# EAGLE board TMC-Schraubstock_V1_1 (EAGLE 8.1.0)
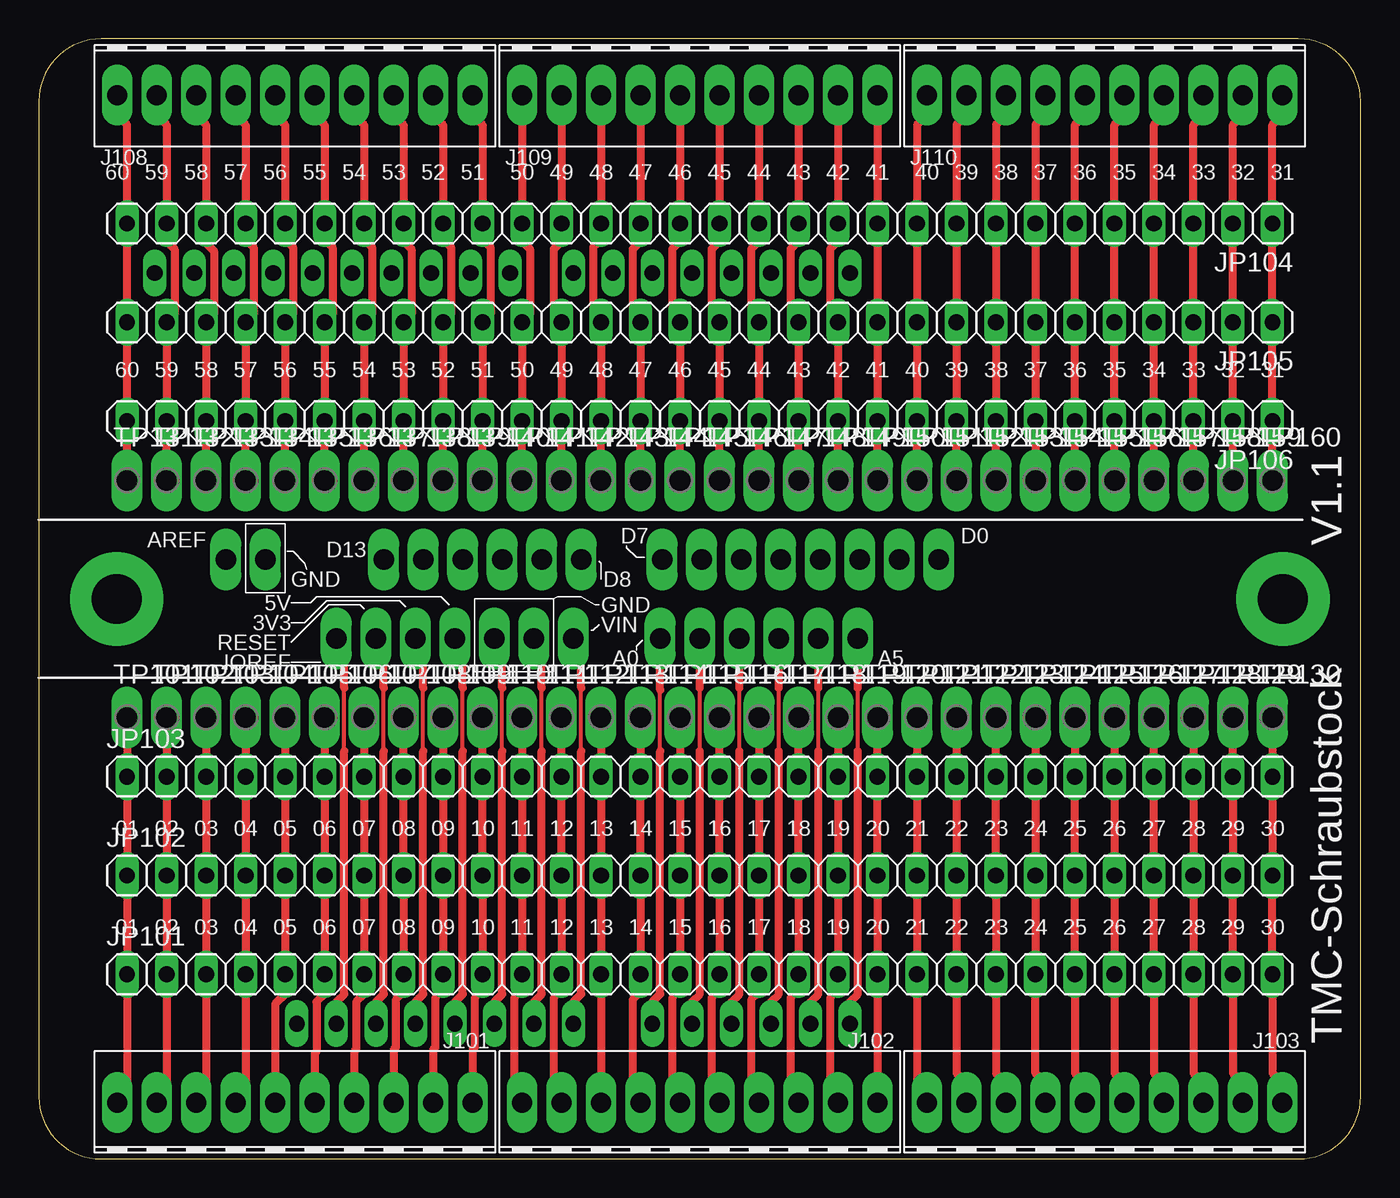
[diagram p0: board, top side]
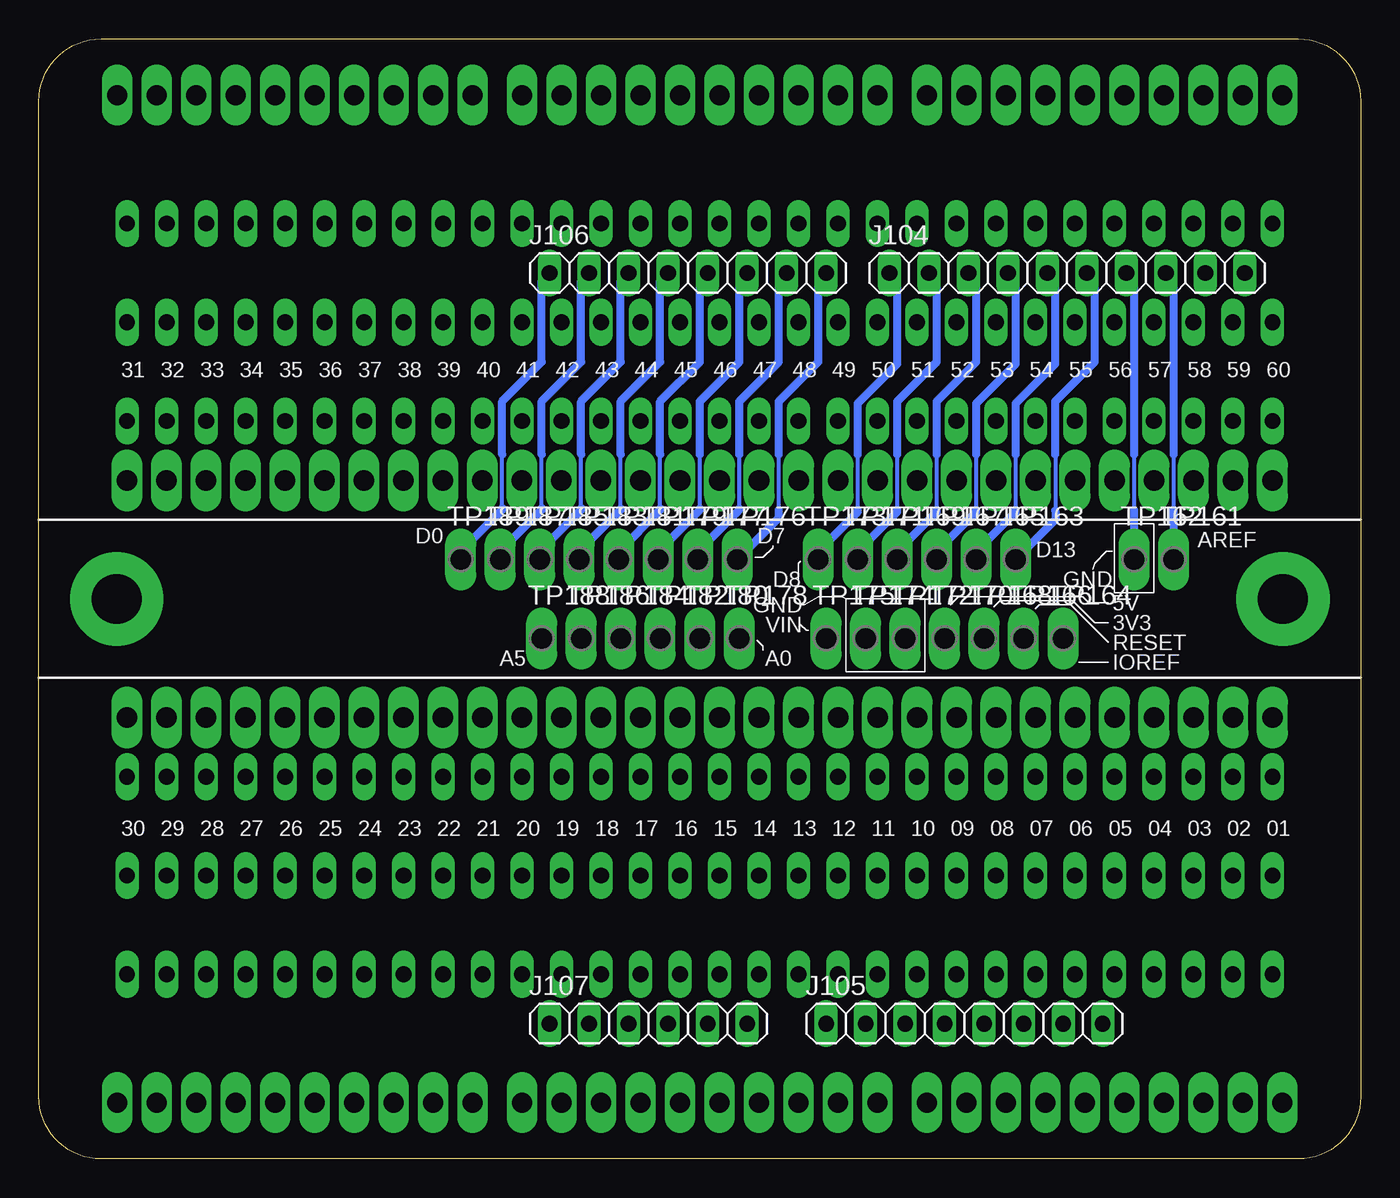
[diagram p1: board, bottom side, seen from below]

Size 85 x 72 mm. Coordinates in mm from the lower left corner, seen from the top.
Outline: 0,68 0,4 arc90 4,0 81,0 arc90 85,4 85,68 arc90 81,72 4,72 arc90 0,68
Copper layers (1*16): Top 0.018mm / dielectric 1.55mm / Bottom 0.018mm
Design rules "eC_2Layer_PClass6_BaseCopperO18_eCDefault": minimum track width 0.15mm, minimum drill 0.35mm, track to track 0.15mm, track to pad 0.15mm, pad to pad 0.15mm, via to via 0.15mm, smd to smd 0mil, copper to edge 0.25mm, drill to drill 0.35mm, minimum pad ring 0.175mm, minimum via ring 0.125mm, stop-mask expansion 0mil, vias tented up to drill 0.45mm, thermal gap 0.2mm

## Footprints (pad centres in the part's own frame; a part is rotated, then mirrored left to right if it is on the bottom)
OSTVN10A150 = drill 1.3 long: 1 -11.43,0; 2 -8.89,0; 3 -6.35,0; 4 -3.81,0; 5 -1.27,0; 6 1.27,0; 7 3.81,0; 8 6.35,0; 9 8.89,0; 10 11.43,0
1X10 = drill 1.016 long: 1 -11.43,0; 2 -8.89,0; 3 -6.35,0; 4 -3.81,0; 5 -1.27,0; 6 1.27,0; 7 3.81,0; 8 6.35,0; 9 8.89,0; 10 11.43,0
1X08 = drill 1.016 long: 1 -8.89,0; 2 -6.35,0; 3 -3.81,0; 4 -1.27,0; 5 1.27,0; 6 3.81,0; 7 6.35,0; 8 8.89,0
1X06 = drill 1.016 long: 1 -6.35,0; 2 -3.81,0; 3 -1.27,0; 4 1.27,0; 5 3.81,0; 6 6.35,0
1X30 = drill 1.016 long: 1 -36.83,0; 2 -34.29,0; 3 -31.75,0; 4 -29.21,0; 5 -26.67,0; 6 -24.13,0; 7 -21.59,0; 8 -19.05,0; 9 -16.51,0; 10 -13.97,0; 11 -11.43,0; 12 -8.89,0; 13 -6.35,0; 14 -3.81,0; 15 -1.27,0; 16 1.27,0; 17 3.81,0; 18 6.35,0; 19 8.89,0; 20 11.43,0; 21 13.97,0; 22 16.51,0; 23 19.05,0; 24 21.59,0; 25 24.13,0; 26 26.67,0; 27 29.21,0; 28 31.75,0; 29 34.29,0; 30 36.83,0
P1-13Y = drill 1.321 pad 1.905 long: TP 0,0

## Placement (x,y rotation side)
J101  [OSTVN10A150]  16.46,3.62 0 top
J102  [OSTVN10A150]  42.5,3.62 0 top
J103  [OSTVN10A150]  68.53,3.62 0 top
J104  PINHD-1X10  [1X10]  18.88,56.95 0 bottom
J105  PINHD-1X8  [1X08]  25.48,8.7 0 bottom
J106  PINHD-1X8  [1X08]  43.26,56.95 0 bottom
J107  PINHD-1X6  [1X06]  45.8,8.7 0 bottom
J108  [OSTVN10A150]  16.46,68.38 180 top
J109  [OSTVN10A150]  42.5,68.38 180 top
J110  [OSTVN10A150]  68.53,68.38 180 top
JP101  [1X30]  42.5,11.87 0 top
JP102  [1X30]  42.5,18.22 0 top
JP103  [1X30]  42.5,24.57 0 top
JP104  [1X30]  42.5,60.13 180 top
JP105  [1X30]  42.5,53.78 180 top
JP106  [1X30]  42.5,47.43 180 top
TP101  TPSPAD1-13Y  [P1-13Y]  5.67,28.38 0 top
TP102  TPSPAD1-13Y  [P1-13Y]  8.21,28.38 0 top
TP103  TPSPAD1-13Y  [P1-13Y]  10.75,28.38 0 top
TP104  TPSPAD1-13Y  [P1-13Y]  13.29,28.38 0 top
TP105  TPSPAD1-13Y  [P1-13Y]  15.83,28.38 0 top
TP106  TPSPAD1-13Y  [P1-13Y]  18.37,28.38 0 top
TP107  TPSPAD1-13Y  [P1-13Y]  20.91,28.38 0 top
TP108  TPSPAD1-13Y  [P1-13Y]  23.45,28.38 0 top
TP109  TPSPAD1-13Y  [P1-13Y]  25.99,28.38 0 top
TP110  TPSPAD1-13Y  [P1-13Y]  28.53,28.38 0 top
TP111  TPSPAD1-13Y  [P1-13Y]  31.07,28.38 0 top
TP112  TPSPAD1-13Y  [P1-13Y]  33.61,28.38 0 top
TP113  TPSPAD1-13Y  [P1-13Y]  36.15,28.38 0 top
TP114  TPSPAD1-13Y  [P1-13Y]  38.69,28.38 0 top
TP115  TPSPAD1-13Y  [P1-13Y]  41.23,28.38 0 top
TP116  TPSPAD1-13Y  [P1-13Y]  43.77,28.38 0 top
TP117  TPSPAD1-13Y  [P1-13Y]  46.31,28.38 0 top
TP118  TPSPAD1-13Y  [P1-13Y]  48.85,28.38 0 top
TP119  TPSPAD1-13Y  [P1-13Y]  51.39,28.38 0 top
TP120  TPSPAD1-13Y  [P1-13Y]  53.93,28.38 0 top
TP121  TPSPAD1-13Y  [P1-13Y]  56.47,28.38 0 top
TP122  TPSPAD1-13Y  [P1-13Y]  59.01,28.38 0 top
TP123  TPSPAD1-13Y  [P1-13Y]  61.55,28.38 0 top
TP124  TPSPAD1-13Y  [P1-13Y]  64.09,28.38 0 top
TP125  TPSPAD1-13Y  [P1-13Y]  66.63,28.38 0 top
TP126  TPSPAD1-13Y  [P1-13Y]  69.17,28.38 0 top
TP127  TPSPAD1-13Y  [P1-13Y]  71.71,28.38 0 top
TP128  TPSPAD1-13Y  [P1-13Y]  74.25,28.38 0 top
TP129  TPSPAD1-13Y  [P1-13Y]  76.79,28.38 0 top
TP130  TPSPAD1-13Y  [P1-13Y]  79.33,28.38 0 top
TP131  TPSPAD1-13Y  [P1-13Y]  5.67,43.62 0 top
TP132  TPSPAD1-13Y  [P1-13Y]  8.21,43.62 0 top
TP133  TPSPAD1-13Y  [P1-13Y]  10.75,43.62 0 top
TP134  TPSPAD1-13Y  [P1-13Y]  13.29,43.62 0 top
TP135  TPSPAD1-13Y  [P1-13Y]  15.83,43.62 0 top
TP136  TPSPAD1-13Y  [P1-13Y]  18.37,43.62 0 top
TP137  TPSPAD1-13Y  [P1-13Y]  20.91,43.62 0 top
TP138  TPSPAD1-13Y  [P1-13Y]  23.45,43.62 0 top
TP139  TPSPAD1-13Y  [P1-13Y]  25.99,43.62 0 top
TP140  TPSPAD1-13Y  [P1-13Y]  28.53,43.62 0 top
TP141  TPSPAD1-13Y  [P1-13Y]  31.07,43.62 0 top
TP142  TPSPAD1-13Y  [P1-13Y]  33.61,43.62 0 top
TP143  TPSPAD1-13Y  [P1-13Y]  36.15,43.62 0 top
TP144  TPSPAD1-13Y  [P1-13Y]  38.69,43.62 0 top
TP145  TPSPAD1-13Y  [P1-13Y]  41.23,43.62 0 top
TP146  TPSPAD1-13Y  [P1-13Y]  43.77,43.62 0 top
TP147  TPSPAD1-13Y  [P1-13Y]  46.31,43.62 0 top
TP148  TPSPAD1-13Y  [P1-13Y]  48.85,43.62 0 top
TP149  TPSPAD1-13Y  [P1-13Y]  51.39,43.62 0 top
TP150  TPSPAD1-13Y  [P1-13Y]  53.93,43.62 0 top
TP151  TPSPAD1-13Y  [P1-13Y]  56.47,43.62 0 top
TP152  TPSPAD1-13Y  [P1-13Y]  59.01,43.62 0 top
TP153  TPSPAD1-13Y  [P1-13Y]  61.55,43.62 0 top
TP154  TPSPAD1-13Y  [P1-13Y]  64.09,43.62 0 top
TP155  TPSPAD1-13Y  [P1-13Y]  66.63,43.62 0 top
TP156  TPSPAD1-13Y  [P1-13Y]  69.17,43.62 0 top
TP157  TPSPAD1-13Y  [P1-13Y]  71.71,43.62 0 top
TP158  TPSPAD1-13Y  [P1-13Y]  74.25,43.62 0 top
TP159  TPSPAD1-13Y  [P1-13Y]  76.79,43.62 0 top
TP160  TPSPAD1-13Y  [P1-13Y]  79.33,43.62 0 top
TP161  TPSPAD1-13Y  [P1-13Y]  12.02,38.54 0 bottom
TP162  TPSPAD1-13Y  [P1-13Y]  14.56,38.54 0 bottom
TP163  TPSPAD1-13Y  [P1-13Y]  22.18,38.54 0 bottom
TP164  TPSPAD1-13Y  [P1-13Y]  19.13,33.46 0 bottom
TP165  TPSPAD1-13Y  [P1-13Y]  24.72,38.54 0 bottom
TP166  TPSPAD1-13Y  [P1-13Y]  21.67,33.46 0 bottom
TP167  TPSPAD1-13Y  [P1-13Y]  27.26,38.54 0 bottom
TP168  TPSPAD1-13Y  [P1-13Y]  24.21,33.46 0 bottom
TP169  TPSPAD1-13Y  [P1-13Y]  29.8,38.54 0 bottom
TP170  TPSPAD1-13Y  [P1-13Y]  26.75,33.46 0 bottom
TP171  TPSPAD1-13Y  [P1-13Y]  32.34,38.54 0 bottom
TP172  TPSPAD1-13Y  [P1-13Y]  29.29,33.46 0 bottom
TP173  TPSPAD1-13Y  [P1-13Y]  34.88,38.54 0 bottom
TP174  TPSPAD1-13Y  [P1-13Y]  31.83,33.46 0 bottom
TP175  TPSPAD1-13Y  [P1-13Y]  34.37,33.46 0 bottom
TP176  TPSPAD1-13Y  [P1-13Y]  40.09,38.54 0 bottom
TP177  TPSPAD1-13Y  [P1-13Y]  42.63,38.54 0 bottom
TP178  TPSPAD1-13Y  [P1-13Y]  39.96,33.46 0 bottom
TP179  TPSPAD1-13Y  [P1-13Y]  45.17,38.54 0 bottom
TP180  TPSPAD1-13Y  [P1-13Y]  42.5,33.46 0 bottom
TP181  TPSPAD1-13Y  [P1-13Y]  47.71,38.54 0 bottom
TP182  TPSPAD1-13Y  [P1-13Y]  45.04,33.46 0 bottom
TP183  TPSPAD1-13Y  [P1-13Y]  50.25,38.54 0 bottom
TP184  TPSPAD1-13Y  [P1-13Y]  47.58,33.46 0 bottom
TP185  TPSPAD1-13Y  [P1-13Y]  52.79,38.54 0 bottom
TP186  TPSPAD1-13Y  [P1-13Y]  50.12,33.46 0 bottom
TP187  TPSPAD1-13Y  [P1-13Y]  55.33,38.54 0 bottom
TP188  TPSPAD1-13Y  [P1-13Y]  52.66,33.46 0 bottom
TP189  TPSPAD1-13Y  [P1-13Y]  57.87,38.54 0 bottom

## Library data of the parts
J101-J110 TP101-TP189 = TMC-Schraubstock
JP101-JP106 = pinhead

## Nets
N$1: J101.1 JP101.1 JP102.1 JP103.1 TP101.TP
N$2: J101.2 JP101.2 JP102.2 JP103.2 TP102.TP
N$3: J101.3 JP101.3 JP102.3 JP103.3 TP103.TP
N$4: J101.4 JP101.4 JP102.4 JP103.4 TP104.TP
N$5: J101.5 JP101.5 JP102.5 JP103.5 TP105.TP
N$6: J101.6 JP101.6 JP102.6 JP103.6 TP106.TP
N$7: J101.7 JP101.7 JP102.7 JP103.7 TP107.TP
N$8: J101.8 JP101.8 JP102.8 JP103.8 TP108.TP
N$9: J101.9 JP101.9 JP102.9 JP103.9 TP109.TP
N$10: J101.10 JP101.10 JP102.10 JP103.10 TP110.TP
N$11: J102.1 JP101.11 JP102.11 JP103.11 TP111.TP
N$12: J102.2 JP101.12 JP102.12 JP103.12 TP112.TP
N$13: J102.3 JP101.13 JP102.13 JP103.13 TP113.TP
N$14: J102.4 JP101.14 JP102.14 JP103.14 TP114.TP
N$15: J102.5 JP101.15 JP102.15 JP103.15 TP115.TP
N$16: J102.6 JP101.16 JP102.16 JP103.16 TP116.TP
N$17: J102.7 JP101.17 JP102.17 JP103.17 TP117.TP
N$18: J102.8 JP101.18 JP102.18 JP103.18 TP118.TP
N$19: J102.9 JP101.19 JP102.19 JP103.19 TP119.TP
N$20: J102.10 JP101.20 JP102.20 JP103.20 TP120.TP
N$21: J103.1 JP101.21 JP102.21 JP103.21 TP121.TP
N$22: J103.2 JP101.22 JP102.22 JP103.22 TP122.TP
N$23: J103.3 JP101.23 JP102.23 JP103.23 TP123.TP
N$24: J103.4 JP101.24 JP102.24 JP103.24 TP124.TP
N$25: J103.5 JP101.25 JP102.25 JP103.25 TP125.TP
N$26: J103.6 JP101.26 JP102.26 JP103.26 TP126.TP
N$27: J103.7 JP101.27 JP102.27 JP103.27 TP127.TP
N$28: J103.8 JP101.28 JP102.28 JP103.28 TP128.TP
N$29: J103.9 JP101.29 JP102.29 JP103.29 TP129.TP
N$30: J103.10 JP101.30 JP102.30 JP103.30 TP130.TP
N$31: J110.1 JP104.1 JP105.1 JP106.1 TP160.TP
N$32: J110.2 JP104.2 JP105.2 JP106.2 TP159.TP
N$33: J110.3 JP104.3 JP105.3 JP106.3 TP158.TP
N$34: J110.4 JP104.4 JP105.4 JP106.4 TP157.TP
N$35: J110.5 JP104.5 JP105.5 JP106.5 TP156.TP
N$36: J110.6 JP104.6 JP105.6 JP106.6 TP155.TP
N$37: J110.7 JP104.7 JP105.7 JP106.7 TP154.TP
N$38: J110.8 JP104.8 JP105.8 JP106.8 TP153.TP
N$39: J110.9 JP104.9 JP105.9 JP106.9 TP152.TP
N$40: J110.10 JP104.10 JP105.10 JP106.10 TP151.TP
N$41: J109.1 JP104.11 JP105.11 JP106.11 TP150.TP
N$42: J109.2 JP104.12 JP105.12 JP106.12 TP149.TP
N$43: J109.3 JP104.13 JP105.13 JP106.13 TP148.TP
N$44: J109.4 JP104.14 JP105.14 JP106.14 TP147.TP
N$45: J109.5 JP104.15 JP105.15 JP106.15 TP146.TP
N$46: J109.6 JP104.16 JP105.16 JP106.16 TP145.TP
N$47: J109.7 JP104.17 JP105.17 JP106.17 TP144.TP
N$48: J109.8 JP104.18 JP105.18 JP106.18 TP143.TP
N$49: J109.9 JP104.19 JP105.19 JP106.19 TP142.TP
N$50: J109.10 JP104.20 JP105.20 JP106.20 TP141.TP
N$51: J108.1 JP104.21 JP105.21 JP106.21 TP140.TP
N$52: J108.2 JP104.22 JP105.22 JP106.22 TP139.TP
N$53: J108.3 JP104.23 JP105.23 JP106.23 TP138.TP
N$54: J108.4 JP104.24 JP105.24 JP106.24 TP137.TP
N$55: J108.5 JP104.25 JP105.25 JP106.25 TP136.TP
N$56: J108.6 JP104.26 JP105.26 JP106.26 TP135.TP
N$57: J108.7 JP104.27 JP105.27 JP106.27 TP134.TP
N$58: J108.8 JP104.28 JP105.28 JP106.28 TP133.TP
N$59: J108.9 JP104.29 JP105.29 JP106.29 TP132.TP
N$60: J108.10 JP104.30 JP105.30 JP106.30 TP131.TP
N$62: J107.1 TP188.TP
N$63: J107.2 TP186.TP
N$64: J107.3 TP184.TP
N$65: J107.4 TP182.TP
N$66: J107.5 TP180.TP
N$67: J107.6 TP178.TP
N$68: J105.1 TP175.TP
N$69: J105.2 TP174.TP
N$70: J105.3 TP172.TP
N$71: J105.4 TP170.TP
N$72: J105.5 TP168.TP
N$73: J105.6 TP166.TP
N$74: J105.7 TP164.TP
N$76: J106.8 TP176.TP
N$77: J106.7 TP177.TP
N$78: J106.6 TP179.TP
N$79: J106.5 TP181.TP
N$80: J106.4 TP183.TP
N$81: J106.3 TP185.TP
N$82: J106.2 TP187.TP
N$83: J106.1 TP189.TP
N$86: J104.8 TP161.TP
N$87: J104.7 TP162.TP
N$88: J104.6 TP163.TP
N$89: J104.5 TP165.TP
N$90: J104.4 TP167.TP
N$91: J104.3 TP169.TP
N$92: J104.2 TP171.TP
N$93: J104.1 TP173.TP

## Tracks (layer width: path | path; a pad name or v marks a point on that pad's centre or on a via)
N$1
  Top 0.508: TP101.TP JP103.1 JP102.1 JP101.1 5.67,4.25 J101.1
N$2
  Top 0.508: TP102.TP JP103.2 JP102.2 JP101.2 8.21,4.25 J101.2
N$3
  Top 0.508: TP103.TP JP103.3 JP102.3 JP101.3 10.75,4.25 J101.3
N$4
  Top 0.508: TP104.TP JP103.4 JP102.4 JP101.4 13.29,4.25 J101.4
N$5
  Top 0.508: TP105.TP JP103.5 JP102.5 JP101.5 | JP101.5 15.83,10.85 | JP101.5 15.83,10.6 15.2,9.96 J101.5
N$6
  Top 0.508: TP106.TP JP103.6 JP102.6 JP101.6 18.37,10.6 17.86,10.09 17.86,6.92 17.73,6.79 J101.6
N$7
  Top 0.508: TP107.TP JP103.7 JP102.7 JP101.7 20.91,10.6 20.4,10.09 20.4,7.04 20.27,6.92 J101.7
N$8
  Top 0.508: TP108.TP JP103.8 JP102.8 JP101.8 23.45,10.73 22.94,10.22 22.94,7.17 22.82,7.04 J101.8
N$9
  Top 0.508: TP109.TP JP103.9 JP102.9 JP101.9 25.99,10.85 25.48,10.35 25.48,7.17 25.36,7.04 J101.9
N$10
  Top 0.508: JP101.10 JP102.10 JP103.10 TP110.TP | JP101.10 28.53,11.74 | JP101.10 28.53,10.85 28.02,10.35 28.02,7.17 27.89,7.04 J101.10
N$11
  Top 0.508: TP111.TP JP103.11 JP102.11 JP101.11 31.07,10.85 30.56,10.35 30.56,4.12 J102.1
N$12
  Top 0.508: TP112.TP JP103.12 JP102.12 JP101.12 33.61,10.85 33.1,10.35 33.1,4.12 J102.2
N$13
  Top 0.508: TP113.TP JP103.13 JP102.13 JP101.13 J102.3
N$14
  Top 0.508: TP114.TP JP103.14 JP102.14 JP101.14 38.69,10.73 38.18,10.22 38.18,4.12 J102.4
N$15
  Top 0.508: TP115.TP JP103.15 41.25,24.55 41.25,18.22 JP102.15 JP101.15 41.23,10.85 40.72,10.35 40.72,4.12 J102.5
N$16
  Top 0.508: TP116.TP JP103.16 JP102.16 JP101.16 43.77,10.85 43.26,10.35 43.26,4.12 J102.6
N$17
  Top 0.508: TP117.TP JP103.17 JP102.17 JP101.17 46.31,10.73 45.8,10.22 45.8,4.12 J102.7
N$18
  Top 0.508: TP118.TP JP103.18 JP102.18 JP101.18 48.85,10.85 48.34,10.35 48.34,4.12 J102.8
N$19
  Top 0.508: TP119.TP JP103.19 JP102.19 JP101.19 51.39,10.85 50.88,10.35 50.88,4.12 J102.9
N$20
  Top 0.508: TP120.TP JP103.20 JP102.20 JP101.20 J102.10
N$21
  Top 0.508: TP121.TP JP103.21 JP102.21 JP101.21 56.47,4.25 J103.1
N$22
  Top 0.508: TP122.TP JP103.22 JP102.22 JP101.22 59.01,5.52 59.64,4.89 J103.2
N$23
  Top 0.508: TP123.TP JP103.23 JP102.23 JP101.23 61.55,5.52 62.19,4.89 J103.3
N$24
  Top 0.508: TP124.TP JP103.24 JP102.24 JP101.24 64.09,5.52 64.72,4.89 J103.4
N$25
  Top 0.508: TP125.TP JP103.25 JP102.25 JP101.25 66.63,5.52 67.27,4.89 J103.5
N$26
  Top 0.508: TP126.TP JP103.26 JP102.26 JP101.26 69.17,5.52 69.81,4.89 J103.6
N$27
  Top 0.508: TP127.TP JP103.27 JP102.27 JP101.27 71.71,5.52 72.34,4.89 J103.7
N$28
  Top 0.508: TP128.TP JP103.28 JP102.28 JP101.28 74.25,5.52 74.88,4.89 J103.8
N$29
  Top 0.508: TP129.TP JP103.29 JP102.29 JP101.29 76.79,5.52 77.42,4.89 J103.9
N$30
  Top 0.508: TP130.TP JP103.30 JP102.30 | JP102.30 79.33,17.59 | JP102.30 JP101.30 79.33,5.52 79.97,4.89 J103.10
N$31
  Top 0.508: TP160.TP JP106.1 JP105.1 JP104.1 79.33,66.48 79.97,67.11 J110.1
N$32
  Top 0.508: TP159.TP JP106.2 JP105.2 JP104.2 76.79,66.48 77.42,67.11 J110.2
N$33
  Top 0.508: TP158.TP JP106.3 JP105.3 JP104.3 74.25,66.48 74.88,67.11 J110.3
N$34
  Top 0.508: TP157.TP JP106.4 JP105.4 JP104.4 71.71,66.48 72.34,67.11 J110.4
N$35
  Top 0.508: TP156.TP JP106.5 JP105.5 JP104.5 69.17,66.48 69.81,67.11 J110.5
N$36
  Top 0.508: TP155.TP JP106.6 JP105.6 JP104.6 66.63,66.48 67.27,67.11 J110.6
N$37
  Top 0.508: TP154.TP JP106.7 JP105.7 JP104.7 64.09,66.48 64.72,67.11 J110.7
N$38
  Top 0.508: TP153.TP JP106.8 JP105.8 JP104.8 61.55,66.48 62.19,67.11 J110.8
N$39
  Top 0.508: TP152.TP JP106.9 JP105.9 JP104.9 59.01,66.48 59.64,67.11 J110.9
N$40
  Top 0.508: TP151.TP JP106.10 JP105.10 JP104.10 56.47,66.48 57.11,67.11 J110.10
N$41
  Top 0.508: J109.1 JP104.11 JP105.11 JP106.11 TP150.TP
N$42
  Top 0.508: J109.2 JP104.12 | TP149.TP JP106.12 JP105.12 50.88,54.29 50.88,58.48 51.39,58.99 JP104.12 | JP104.12 51.39,59.88
N$43
  Top 0.508: J109.3 JP104.13 | TP148.TP JP106.13 JP105.13 48.34,54.29 48.34,58.48 48.85,58.99 JP104.13 | JP104.13 48.85,60
N$44
  Top 0.508: J109.4 JP104.14 46.31,58.99 45.8,58.48 45.8,54.29 JP105.14 JP106.14 TP147.TP
N$45
  Top 0.508: TP146.TP JP106.15 JP105.15 43.26,54.29 43.26,58.48 43.77,58.99 JP104.15 J109.5
N$46
  Top 0.508: TP145.TP JP106.16 JP105.16 40.72,54.29 40.72,58.48 41.23,58.99 JP104.16 J109.6
N$47
  Top 0.508: TP144.TP JP106.17 JP105.17 38.18,54.29 38.18,58.48 38.69,58.99 JP104.17 | J109.7 JP104.17 | JP104.17 38.69,59.75
N$48
  Top 0.508: TP143.TP JP106.18 JP105.18 35.64,54.29 35.64,58.61 36.15,59.11 JP104.18 J109.8
N$49
  Top 0.508: TP142.TP JP106.19 JP105.19 33.1,54.29 33.1,58.48 33.61,58.99 JP104.19 J109.9
N$50
  Top 0.508: TP141.TP JP106.20 JP105.20 31.58,54.29 31.58,58.48 31.07,58.99 JP104.20 J109.10
N$51
  Top 0.508: TP140.TP JP106.21 JP105.21 29.04,54.29 29.04,58.61 28.53,59.11 JP104.21 28.53,66.48 27.89,67.11 J108.1
N$52
  Top 0.508: TP139.TP JP106.22 JP105.22 26.5,54.29 26.5,58.61 25.99,59.11 JP104.22 25.99,66.48 25.36,67.11 J108.2
N$53
  Top 0.508: TP138.TP JP106.23 JP105.23 23.96,54.29 23.96,58.48 23.45,58.99 JP104.23 23.45,66.48 22.82,67.11 J108.3
N$54
  Top 0.508: TP137.TP JP106.24 JP105.24 21.42,54.29 21.42,58.61 20.91,59.11 JP104.24 20.91,66.48 20.27,67.11 J108.4
N$55
  Top 0.508: TP136.TP JP106.25 JP105.25 18.88,54.29 18.88,58.61 18.37,59.11 JP104.25 18.37,66.48 17.73,67.11 J108.5
N$56
  Top 0.508: TP135.TP JP106.26 JP105.26 16.34,54.29 16.34,58.61 15.83,59.11 JP104.26 15.83,66.48 15.2,67.11 J108.6
N$57
  Top 0.508: TP134.TP JP106.27 JP105.27 13.8,54.29 13.8,58.61 13.29,59.11 JP104.27 13.29,66.48 12.66,67.11 J108.7
N$58
  Top 0.508: TP133.TP JP106.28 JP105.28 11.26,54.29 11.26,58.35 10.75,58.86 JP104.28 10.75,66.48 10.12,67.11 J108.8
N$59
  Top 0.508: TP132.TP JP106.29 JP105.29 8.72,54.29 8.72,58.48 8.21,58.99 JP104.29 8.21,66.48 7.58,67.11 J108.9
N$60
  Top 0.508: TP131.TP JP106.30 JP105.30 JP104.30 5.67,66.48 5.03,67.11 J108.10
N$61  (via drill 3.2 pad 6)
  other vias: 5,36
N$62
  Top 0.254: 52.66,26.22 52.66,30.29
  Top 0.508: J107.1 52.15,10.09 52.66,10.6 52.66,26.22 | 52.66,30.29 TP188.TP
N$63
  Top 0.254: 50.12,26.22 50.12,30.29
  Top 0.508: J107.2 49.61,10.09 50.12,10.6 50.12,26.22 | 50.12,30.29 TP186.TP
N$64
  Top 0.254: 47.58,26.22 47.58,30.29
  Top 0.508: J107.3 47.07,10.09 47.58,10.6 47.58,26.22 | 47.58,30.29 TP184.TP
N$65
  Top 0.254: 45.04,26.22 45.04,30.29
  Top 0.508: J107.4 44.53,10.09 45.04,10.6 45.04,26.22 | 45.04,30.29 TP182.TP
N$66
  Top 0.254: 42.5,26.22 42.5,30.29
  Top 0.508: J107.5 41.99,10.09 42.5,10.6 42.5,26.22 | 42.5,30.29 TP180.TP
N$67
  Top 0.254: 39.96,26.22 39.96,30.16
  Top 0.508: J107.6 39.45,10.09 39.96,10.6 39.96,26.22 | 39.96,30.16 TP178.TP
N$68
  Top 0.254: 34.88,26.22 34.88,30.29
  Top 0.508: J105.1 34.37,10.09 34.88,10.6 34.88,26.22 | 34.88,30.29 34.88,33.08 TP175.TP
N$69
  Top 0.254: 32.34,26.22 32.34,30.29
  Top 0.508: J105.2 31.83,10.09 32.34,10.6 32.34,26.22 | TP174.TP 32.34,33.08 32.34,30.29
N$70
  Top 0.254: 29.8,26.22 29.8,30.29
  Top 0.508: J105.3 29.29,10.09 29.8,10.6 29.8,26.22 | TP172.TP 29.8,33.08 29.8,30.29
N$71
  Top 0.254: 27.26,26.22 27.26,30.29
  Top 0.508: J105.4 26.75,10.09 27.26,10.6 27.26,26.22 | TP170.TP 27.26,33.08 27.26,30.29
N$72
  Top 0.254: 24.72,26.22 24.72,30.29
  Top 0.508: J105.5 24.21,10.09 24.72,10.6 24.72,26.22 | TP168.TP 24.72,33.08 24.72,30.29
N$73
  Top 0.254: 22.18,26.22 22.18,30.29
  Top 0.508: J105.6 21.67,10.09 22.18,10.6 22.18,26.22 | 22.18,30.29 22.18,33.08 TP166.TP
N$74
  Top 0.254: 19.64,26.22 19.64,30.29
  Top 0.508: J105.7 19.13,10.09 19.64,10.6 19.64,26.22 | 19.64,30.29 19.64,33.08 TP164.TP
N$76
  Bottom 0.254: 37.42,41.72 37.42,45.27
  Bottom 0.508: TP176.TP 37.42,41.21 37.42,41.72 | 37.42,45.27 37.42,48.7 34.88,51.24 34.88,56.45 J106.8
N$77
  Bottom 0.254: 39.96,41.72 39.96,45.27
  Bottom 0.508: TP177.TP 42.63,39.05 39.96,41.72 39.96,41.8 | 39.96,45.27 39.96,48.7 37.42,51.24 37.42,56.45 J106.7
N$78
  Bottom 0.254: 42.5,41.72 42.5,45.27
  Bottom 0.508: TP179.TP 45.17,39.05 42.5,41.72 42.5,41.8 | 42.5,45.27 42.5,48.7 39.96,51.24 39.96,56.45 J106.6
N$79
  Bottom 0.254: 45.04,41.72 45.04,45.27
  Bottom 0.508: TP181.TP 47.71,39.05 45.04,41.72 45.04,41.8 | 45.04,45.27 45.04,48.7 42.5,51.24 42.5,56.45 J106.5
N$80
  Bottom 0.254: 47.58,41.72 47.58,45.27
  Bottom 0.508: TP183.TP 50.25,39.05 47.58,41.72 47.58,41.8 | 47.58,45.27 47.58,48.7 45.04,51.24 45.04,56.45 J106.4
N$81
  Bottom 0.254: 50.12,41.84 50.12,45.27
  Bottom 0.508: TP185.TP 52.79,39.05 50.12,41.72 50.12,41.84 | 50.12,45.27 50.12,48.7 47.58,51.24 47.58,56.45 J106.3
N$82
  Bottom 0.254: 52.66,41.84 52.66,45.27
  Bottom 0.508: TP187.TP 55.33,39.05 52.66,41.72 52.66,41.84 | 52.66,45.27 52.66,48.7 50.12,51.24 50.12,56.45 J106.2
N$83
  Bottom 0.254: 55.2,41.84 55.2,45.27
  Bottom 0.508: TP189.TP 57.87,39.05 55.2,41.72 55.2,41.84 | 55.2,45.27 55.2,48.7 52.66,51.24 52.66,56.45 J106.1
N$86
  Bottom 0.254: 12.02,41.72 12.02,45.27
  Bottom 0.508: TP161.TP 12.02,41.72 | 12.02,45.27 12.02,56.45 J104.8
N$87
  Bottom 0.254: 14.56,41.72 14.56,45.27
  Bottom 0.508: TP162.TP 14.56,41.72 | 14.56,45.27 14.56,56.45 J104.7
N$88
  Bottom 0.254: 19.64,45.27 19.64,41.67
  Bottom 0.508: 19.64,45.27 19.64,48.7 17.1,51.24 17.1,56.45 J104.6 | TP163.TP 19.64,41.08 19.64,41.67
N$89
  Bottom 0.254: 22.18,41.72 22.18,45.27
  Bottom 0.508: TP165.TP 24.72,39.05 22.18,41.59 22.18,41.72 | 22.18,45.27 22.18,48.57 19.64,51.11 19.64,56.45 J104.5
N$90
  Bottom 0.254: 24.72,41.72 24.72,45.27
  Bottom 0.508: TP167.TP 27.26,39.05 24.72,41.59 24.72,41.72 | 24.72,45.27 24.72,48.57 22.18,51.11 22.18,56.45 J104.4
N$91
  Bottom 0.254: 27.26,41.72 27.26,45.27
  Bottom 0.508: TP169.TP 29.8,39.05 27.26,41.59 27.26,41.72 | 27.26,45.27 27.26,48.7 24.72,51.24 24.72,56.45 J104.3
N$92
  Bottom 0.254: 29.8,41.72 29.8,45.27
  Bottom 0.508: TP171.TP 32.34,39.05 29.8,41.59 29.8,41.72 | 29.8,45.27 29.8,48.7 27.26,51.24 27.26,56.45 J104.2
N$93
  Bottom 0.254: 32.34,41.72 32.34,45.27
  Bottom 0.508: TP173.TP 34.88,39.05 32.34,41.59 32.34,41.72 | 32.34,45.27 32.34,48.57 29.8,51.11 29.8,56.45 J104.1
N$94  (via drill 3.2 pad 6)
  other vias: 80,36

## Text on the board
tPlace: 60 | 59 | 58 | 57 | 56 | 55 | 54 | 53 | 52 | 51 | 50 | 49 | 48 | 47 | 46 | 45 | 44 | 43 | 42 | 41 | 40 | 39 | 38 | 37 | 36 | 35 | 34 | 33 | 32 | 31 | 60 | 59 | 58 | 57 | 56 | 55 | 54 | 53 | 52 | 51 | 50 | 49 | 48 | 47 | 46 | 45 | 44 | 43 | 42 | 41 | 40 | 39 | 38 | 37 | 36 | 35 | 34 | 33 | 32 | 31 | V1.1 | AREF | D7 | D0 | D13 | GND | D8 | 5V | GND | 3V3 | VIN | RESET | IOREF | A0 | A5 | 01 | 02 | 03 | 04 | 05 | 06 | 07 | 08 | 09 | 10 | 11 | 12 | 13 | 14 | 15 | 16 | 17 | 18 | 19 | 20 | 21 | 22 | 23 | 24 | 25 | 26 | 27 | 28 | 29 | 30 | TMC-Schraubstock | 01 | 02 | 03 | 04 | 05 | 06 | 07 | 08 | 09 | 10 | 11 | 12 | 13 | 14 | 15 | 16 | 17 | 18 | 19 | 20 | 21 | 22 | 23 | 24 | 25 | 26 | 27 | 28 | 29 | 30
bPlace: 60 | 59 | 58 | 57 | 56 | 55 | 54 | 53 | 52 | 51 | 50 | 49 | 48 | 47 | 46 | 45 | 44 | 43 | 42 | 41 | 40 | 39 | 38 | 37 | 36 | 35 | 34 | 33 | 32 | 31 | AREF | D7 | D0 | D13 | GND | D8 | 5V | GND | 3V3 | VIN | RESET | IOREF | A0 | A5 | 01 | 02 | 03 | 04 | 05 | 06 | 07 | 08 | 09 | 10 | 11 | 12 | 13 | 14 | 15 | 16 | 17 | 18 | 19 | 20 | 21 | 22 | 23 | 24 | 25 | 26 | 27 | 28 | 29 | 30
Measures: (900 mil) | (1400 mil) | (1900 mil)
